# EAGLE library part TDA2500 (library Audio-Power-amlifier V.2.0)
The TDA2500 is a two-channel Amplifier Driver IC that uses Tripath’s proprietary Digital Power Processing (DPPTM) technology. Class-T amplifiers offer both the audio fidelity of Class-AB and the power efficiency of Class-D amplifiers.
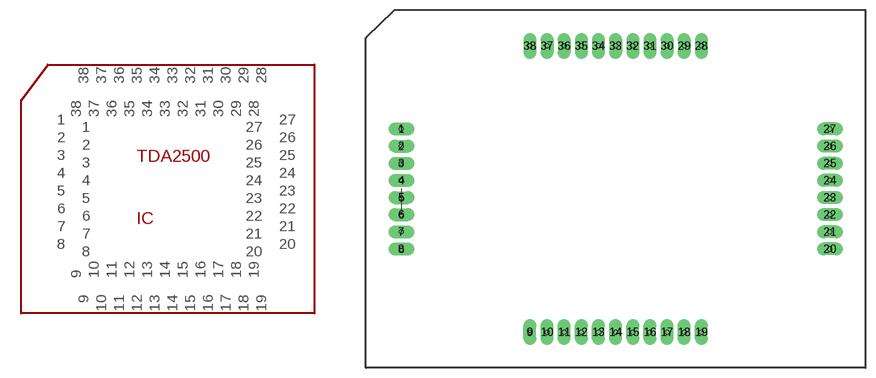
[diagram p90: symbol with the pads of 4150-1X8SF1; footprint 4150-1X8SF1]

Designator prefix IC

## TDA2500  [4150-1X8SF1]
1  1  pwr
2  2
3  3  pwr
4  4
5  5  in
6  6  in
7  7
8  8
9  9  out
10  10  out
11  11
12  12
13  13
14  14
15  15
16  16
17  17
18  18
19  19
20  20  out
21  21
22  22
23  23  pwr
24  24  pwr
25  25
26  26
27  27  out
28  28  pwr
29  29
30  30
31  31
32  32
33  33
34  34
35  35
36  36  nc
37  37  pwr
38  38  pwr

## Footprint 4150-1X8SF1 (pad centres in mm)
drill 0.9 pad 1.93 long: 1 -31.75,8.89; 2 -31.75,6.35; 3 -31.75,3.81; 4 -31.75,1.27; 5 -31.75,-1.27; 6 -31.75,-3.81; 7 -31.75,-6.35; 8 -31.75,-8.89; 9 -12.7,-21.2; 10 -10.16,-21.2; 11 -7.62,-21.2; 12 -5.08,-21.2; 13 -2.54,-21.2; 14 0,-21.2; 15 2.54,-21.2; 16 5.08,-21.2; 17 7.62,-21.2; 18 10.16,-21.2; 19 12.7,-21.2; 20 31.75,-8.89; 21 31.75,-6.35; 22 31.75,-3.81; 23 31.75,-1.27; 24 31.75,1.27; 25 31.75,3.81; 26 31.75,6.35; 27 31.75,8.89; 28 12.7,21.2; 29 10.16,21.2; 30 7.62,21.2; 31 5.08,21.2; 32 2.54,21.2; 33 0,21.2; 34 -2.54,21.2; 35 -5.08,21.2; 36 -7.62,21.2; 37 -10.16,21.2; 38 -12.7,21.2
hole 0.6 at -31.75,8.89
hole 0.6 at -31.75,6.35
hole 0.6 at -31.75,3.81
hole 0.6 at -31.75,1.27
hole 0.6 at -31.75,-1.27
hole 0.6 at -31.75,-3.81
hole 0.6 at -31.75,-6.35
hole 0.6 at -31.75,-8.89
hole 0.6 at 31.75,8.89
hole 0.6 at 31.75,6.35
hole 0.6 at 31.75,3.81
hole 0.6 at 31.75,1.27
hole 0.6 at 31.75,-1.27
hole 0.6 at 31.75,-3.81
hole 0.6 at 31.75,-6.35
hole 0.6 at 31.75,-8.89
hole 0.6 at -12.7,21.2
hole 0.6 at -10.16,21.2
hole 0.6 at -7.62,21.2
hole 0.6 at -5.08,21.2
hole 0.6 at -2.54,21.2
hole 0.6 at 0,21.2
hole 0.6 at 2.54,21.2
hole 0.6 at 5.08,21.2
hole 0.6 at 7.62,21.2
hole 0.6 at 10.16,21.2
hole 0.6 at 12.7,21.2
hole 0.6 at 12.7,-21.2
hole 0.6 at 10.16,-21.2
hole 0.6 at 7.62,-21.2
hole 0.6 at 5.08,-21.2
hole 0.6 at 2.54,-21.2
hole 0.6 at 0,-21.2
hole 0.6 at -2.54,-21.2
hole 0.6 at -5.08,-21.2
hole 0.6 at -7.62,-21.2
hole 0.6 at -10.16,-21.2
hole 0.6 at -12.7,-21.2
